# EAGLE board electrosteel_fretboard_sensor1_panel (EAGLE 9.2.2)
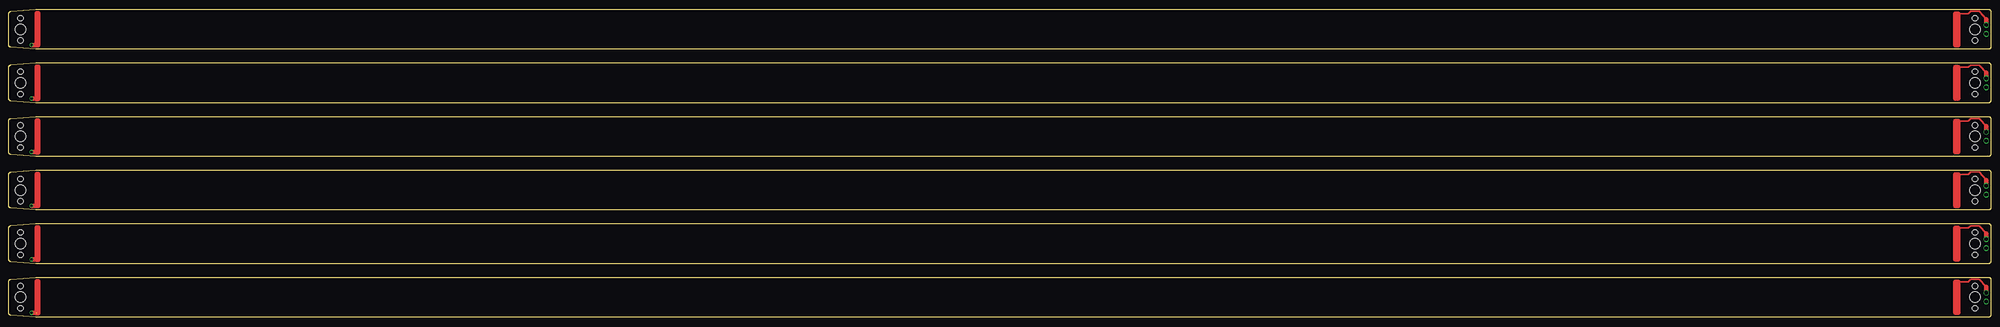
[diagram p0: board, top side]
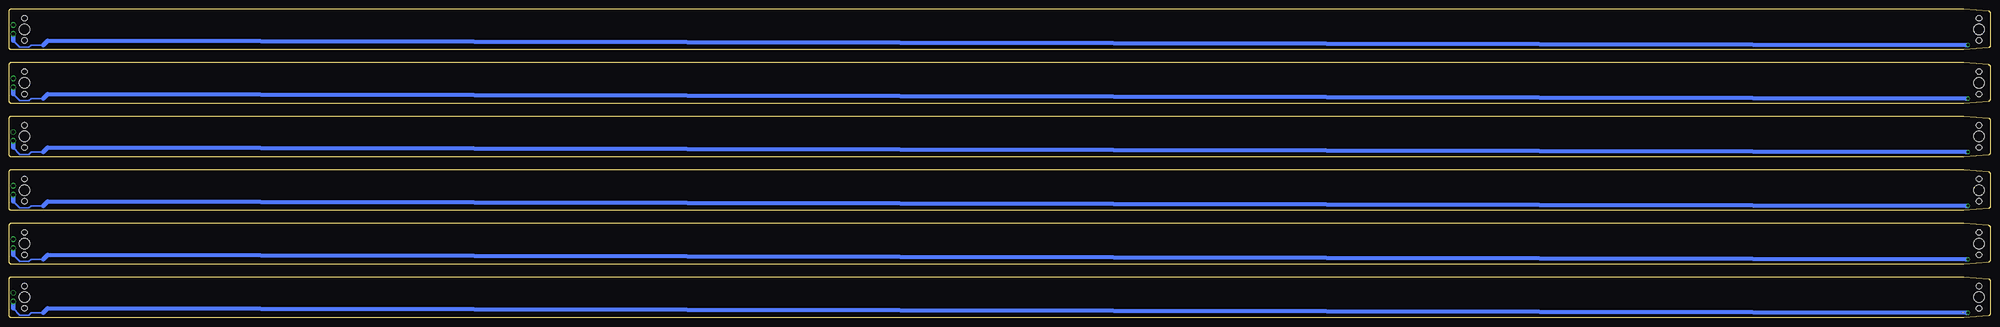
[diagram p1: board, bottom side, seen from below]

Size 562.99 x 87.63 mm. Coordinates in mm from the lower left corner, seen from the top.
Outline: 72 segments
Copper layers (1*16): Top 0.035mm / dielectric 1.5mm / Bottom 0.035mm
Design rules "default *": minimum track width 10mil, minimum drill 24mil, track to track 8mil, track to pad 8mil, pad to pad 8mil, via to via 8mil, smd to smd 8mil, copper to edge 40mil, drill to drill 8mil, minimum pad ring 2mil, minimum via ring 8mil, stop-mask expansion 4mil, vias tented up to drill 0mil, thermal gap 10mil
Holes 3.05 mm at 558.55,5.71 3.3,5.71 558.55,20.95 3.3,20.95 558.55,36.2 3.3,36.2 558.55,51.44 3.3,51.44 558.55,66.67 3.3,66.67 558.55,81.92 3.3,81.92
Holes 1.52 mm at 558.55,8.89 558.55,2.54 3.3,8.89 3.3,2.54 558.55,24.13 558.55,17.78 3.3,24.13 3.3,17.78 558.55,39.37 558.55,33.02 3.3,39.37 3.3,33.02 558.55,54.61 558.55,48.26 3.3,54.61 3.3,48.26 558.55,69.85 558.55,63.5 3.3,69.85 3.3,63.5 558.55,85.09 558.55,78.74 3.3,85.09 3.3,78.74

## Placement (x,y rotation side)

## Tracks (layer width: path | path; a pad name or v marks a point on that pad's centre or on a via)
N$1  (via drill 1.02)
  Top 0.406: 561.72,8.64 559.76,10.79 557.28,10.79 556.64,10.16 553.85,10.16
  Top 1.27: 552.96,10.16 553.72,10.16 553.72,1.27 552.96,1.27 552.96,10.03 | 561.72,8.64 v561.72,6.99
N$2  (via drill 1.02)
  Top 0.406: 561.72,23.88 559.76,26.04 557.28,26.04 556.64,25.4 553.85,25.4
  Top 1.27: 552.96,25.4 553.72,25.4 553.72,16.51 552.96,16.51 552.96,25.27 | 561.72,23.88 v561.72,22.23
N$3  (via drill 1.02)
  Top 0.406: 561.72,39.12 559.76,41.27 557.28,41.27 556.64,40.64 553.85,40.64
  Top 1.27: 552.96,40.64 553.72,40.64 553.72,31.75 552.96,31.75 552.96,40.51 | 561.72,39.12 v561.72,37.47
N$4  (via drill 1.02)
  Top 0.406: 561.72,54.36 559.76,56.52 557.28,56.52 556.64,55.88 553.85,55.88
  Top 1.27: 552.96,55.88 553.72,55.88 553.72,46.99 552.96,46.99 552.96,55.75 | 561.72,54.36 v561.72,52.7
N$5  (via drill 1.02)
  Top 0.406: 561.72,69.6 559.76,71.75 557.28,71.75 556.64,71.12 553.85,71.12
  Top 1.27: 552.96,71.12 553.72,71.12 553.72,62.23 552.96,62.23 552.96,70.99 | 561.72,69.6 v561.72,67.94
N$6  (via drill 1.02)
  Top 0.406: 561.72,84.84 559.76,87 557.28,87 556.64,86.36 553.85,86.36
  Top 1.27: 552.96,86.36 553.72,86.36 553.72,77.47 552.96,77.47 552.96,86.23 | 561.72,84.84 v561.72,83.19
S$1  (via drill 0.65, 1.02)
  Top 1.27: v6.48,16.51 7.75,16.51 | 7.87,16.51 7.87,25.53 8.38,25.53 8.38,16.38 7.75,16.38
  Bottom 0.406: 561.72,17.78 559.82,15.88 557.28,15.88 556.64,16.51 553.21,16.51
  Bottom 1.27: 553.21,16.51 551.95,17.78 7.11,16.51 v6.48,16.51 | 561.72,17.78 v561.72,19.68
S$2  (via drill 0.65, 1.02)
  Top 1.27: v6.48,31.75 7.75,31.75 | 7.87,31.75 7.87,40.77 8.38,40.77 8.38,31.62 7.75,31.62
  Bottom 0.406: 561.72,33.02 559.82,31.11 557.28,31.11 556.64,31.75 553.21,31.75
  Bottom 1.27: 553.21,31.75 551.95,33.02 7.11,31.75 v6.48,31.75 | 561.72,33.02 v561.72,34.92
S$3  (via drill 0.65, 1.02)
  Top 1.27: v6.48,46.99 7.75,46.99 | 7.87,46.99 7.87,56.01 8.38,56.01 8.38,46.86 7.75,46.86
  Bottom 0.406: 561.72,48.26 559.82,46.35 557.28,46.35 556.64,46.99 553.21,46.99
  Bottom 1.27: 553.21,46.99 551.95,48.26 7.11,46.99 v6.48,46.99 | 561.72,48.26 v561.72,50.16
S$4  (via drill 0.65, 1.02)
  Top 1.27: v6.48,62.23 7.75,62.23 | 7.87,62.23 7.87,71.25 8.38,71.25 8.38,62.1 7.75,62.1
  Bottom 0.406: 561.72,63.5 559.82,61.59 557.28,61.59 556.64,62.23 553.21,62.23
  Bottom 1.27: 553.21,62.23 551.95,63.5 7.11,62.23 v6.48,62.23 | 561.72,63.5 v561.72,65.41
S$5  (via drill 0.65, 1.02)
  Top 1.27: v6.48,77.47 7.75,77.47 | 7.87,77.47 7.87,86.49 8.38,86.49 8.38,77.34 7.75,77.34
  Bottom 0.406: 561.72,78.74 559.82,76.83 557.28,76.83 556.64,77.47 553.21,77.47
  Bottom 1.27: 553.21,77.47 551.95,78.74 7.11,77.47 v6.48,77.47 | 561.72,78.74 v561.72,80.64
S$26  (via drill 0.65, 1.02)  (1 unrouted)
  Top 1.27: v6.48,1.27 7.75,1.27 | 7.87,1.27 7.87,10.29 8.38,10.29 8.38,1.14 7.75,1.14
  Bottom 0.406: 561.72,2.54 559.82,0.64 557.28,0.64 556.64,1.27 553.21,1.27
  Bottom 1.27: 553.21,1.27 551.95,2.54 7.11,1.27 v6.48,1.27 | 561.72,2.54 v561.72,4.45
